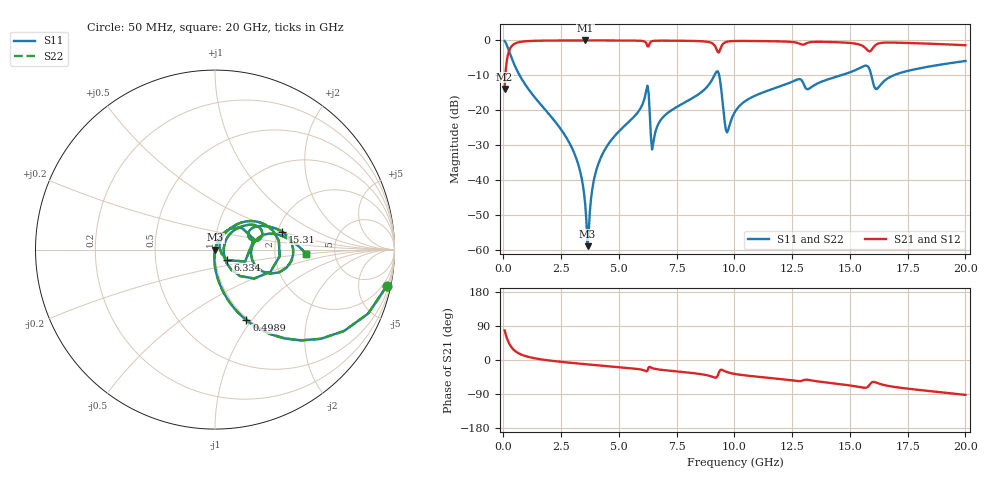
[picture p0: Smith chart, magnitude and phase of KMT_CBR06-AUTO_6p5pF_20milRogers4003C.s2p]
! Data measured by Modelithics Inc. support@modelithics.com 813-866-6335
! KEMET CBR06-AUTO 6.5pF, Pad Width= 0.851mm, Pad Length= 0.64mm, Pad Gap= 0.62mm, 20mil Rogers 4003C substrate Data, January 2022
# hz S ma R 50
! 2 Port Network Data from SP1.SP block
! freq  magS11  angS11  magS21  angS21  magS12  angS12  magS22  angS22
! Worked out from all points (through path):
!   401 points, 50 MHz to 20 GHz, reference 50 ohm
!   highest |S21| = -0.01 dB at 3.541 GHz (marker M1); lowest = -13.9 dB at 50 MHz (marker M2)
!   group delay of S21, straight-line fit = 14.2 ps
!   lowest |S11| = -58.8 dB at 3.641 GHz (marker M3), VSWR 1.00, Z = 50.1 - j0.0651 ohm
!   |S11| at or under -10 dB: 702.2 MHz to 9.131 GHz (8.429 GHz wide, 171 % of centre); 9.339 GHz to 14.6 GHz (5.257 GHz wide, 43.9 % of centre); 15.93 GHz to 16.88 GHz (955 MHz wide, 5.82 % of centre)
!   |S22| runs from -58.8 to -0.2 dB; largest |S21 - S12| = 0
!   S11 on the Smith chart (normalised r, x): 50 MHz: 0.98, -9.57; 498.9 MHz: 0.98, -0.94; 6.334 GHz: 1.14, -0.14; 15.31 GHz: 2.11, +0.50; 20 GHz: 3.05, -0.20
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5e7  0.9794 -11.8  0.2019 78.2  0.2019 78.2  0.9794 -11.8
4.98875e8  0.4309 -66.0  0.9018 23.9  0.9018 23.9  0.4309 -66.0
2.74325e9  0.03996 -95.1  0.9982 -6.4  0.9982 -6.4  0.03996 -95.1
3.391625e9  0.0105 -94.6  0.9988 -10.2  0.9988 -10.2  0.0105 -94.6
3.54125e9  0.004506 -87.6  0.9988 -11.0  0.9988 -11.0  0.004506 -87.6
3.641e9  0.001149 -34.5  0.9988 -11.5  0.9988 -11.5  0.001149 -34.5
3.990125e9  0.01288 71.6  0.9987 -13.4  0.9987 -13.4  0.01288 71.6
4.389125e9  0.02748 72.0  0.9983 -15.5  0.9983 -15.5  0.02748 72.0
6.184625e9  0.1926 38.4  0.9124 -29.9  0.9124 -29.9  0.1926 38.4
6.33425e9  0.091 -40.5  0.9151 -18.1  0.9151 -18.1  0.091 -40.5
6.483875e9  0.03332 39.4  0.9835 -22.2  0.9835 -22.2  0.03332 39.4
6.73325e9  0.06666 60.3  0.9922 -25.1  0.9922 -25.1  0.06666 60.3
9.227e9  0.3591 8.0  0.7451 -45.9  0.7451 -45.9  0.3591 8.0
9.675875e9  0.0485 -1.3  0.9576 -31.8  0.9576 -31.8  0.0485 -1.3
1.0025e10  0.09562 44.4  0.9807 -36.9  0.9807 -36.9  0.09562 44.4
1.271825e10  0.2765 26.5  0.9236 -55.6  0.9236 -55.6  0.2765 26.5
1.336662e10  0.2191 28.9  0.9494 -54.3  0.9494 -54.3  0.2191 28.9
1.531175e10  0.3862 15.0  0.8902 -70.2  0.8902 -70.2  0.3862 15.0
1.591025e10  0.3348 -23.6  0.7131 -61.1  0.7131 -61.1  0.3348 -23.6
1.615962e10  0.202 -0.7  0.8815 -60.1  0.8815 -60.1  0.202 -0.7
1.670825e10  0.2964 16.8  0.9325 -68.9  0.9325 -68.9  0.2964 16.8
2e10  0.5084 -2.8  0.8538 -92.0  0.8538 -92.0  0.5084 -2.8
